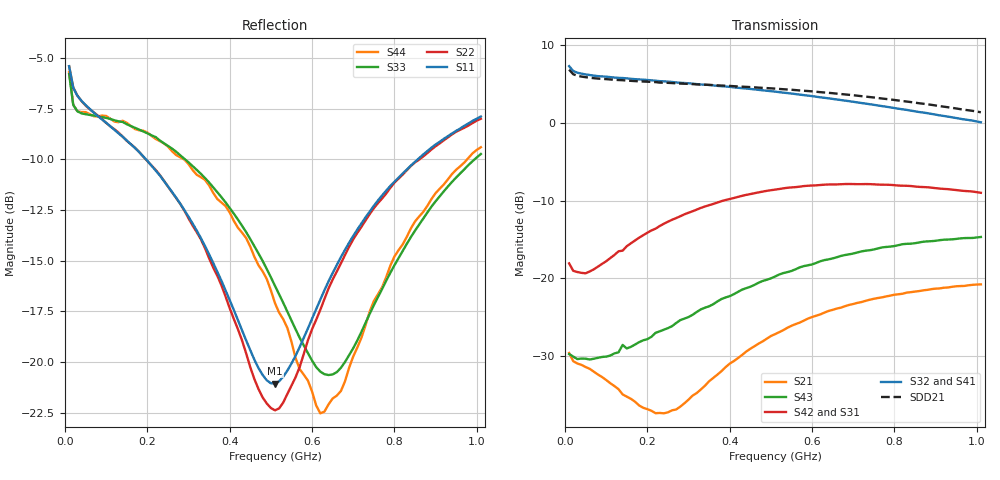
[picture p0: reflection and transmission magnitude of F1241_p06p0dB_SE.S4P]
! Integrated Device Technology
! Corporate Headquarters
! 6024 Silver Creek Valley Road
! San Jose, CA 95138  USA
! Phone:  1-408-284-8200
! Toll Free:  1-800-223-1366
! Webpage:  http://www.idt.com/
! Timing and RF Division
! 515 Groton Road, Suite 102
! Westford, MA 01886-6024
! Device:  F1241
! Description: Dual Intermediate Frequency Digital Variable Gain Amplifier
! Frequency:  10.0 -  500.00 MHz
! Package:  5x5 mm QFN Plastic Package: 32 pin
! Ports:  8 RF, 20 DC
!  Pin  1  = GA3  Pin 17  = RF OUT_B+
!  Pin  2  = GA4  Pin 18  = RF OUT_B-
!  Pin  3  = GA5  Pin 19  = STBY_B
!  Pin  4  = ISET_A  Pin 20  = Ground
!  Pin  5  = ISET_B  Pin 21  = Ground
!  Pin  6  = GB5  Pin 22  = STB_A
!  Pin  7  = GB4  Pin 23  = RF OUT_A-  = Port 4
!  Pin  8  = GB3  Pin 24  = RF OUT_A+  = Port 3
!  Pin  9  = GB2  Pin 25  = NO CONNECT
!  Pin 10  = GB1  Pin 26  = NO CONNECT
!  Pin 11  = RF IN_B+  Pin 27  = VCC
!  Pin 12  = RF IN_B-  Pin 28  = Ground
!  Pin 13  = Ground  Pin 29  = RF IN_A-  = Port 2
!  Pin 14  = VCC  Pin 30  = RF IN_A+  = Port 1
!  Pin 15  = NO CONNECT  Pin 31  = GA1
!  Pin 16  = NO CONNECT  Pin 32  = GA2
! State:  14
! Gain State:  6.0 dB
! Voltages:  Vcc = +5.00 Volts  Icc approximately 160.0 mA or 80 mA per channel.
! Data:  The device was measured on a custom evaluation board which has
!  individual transmission lines to the RF pins.  Data was collected
!  using a calibrated network analyzer.  The evaluation board was
!  de-embedded using a port reference technique.
!  The reference plane is the edge of the package pin.
!  Only Channel A was measured.
!  This data is in single-ended operation.  If your needs are balanced
!  or differential S-parameters then this file needs to be used a
!  linear simulator.
! Misc:  Lot Code  160028MY
!  Action Tracker AT004
! Date Measured:  2014-08-14
! Date:  2014-08-28  MJV
! Note:
!  Integrated Device Technology supplies this data as a sample of measured
!  data at the package pin for this product.  Your particular data for this
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# Hz S dB R 50
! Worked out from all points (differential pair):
!   101 points, 10 MHz to 1.01 GHz, reference 50 ohm
!   strongest paths, dB at 10 MHz, 260 MHz, 510 MHz, 760 MHz, 1.01 GHz:
!     S32: 7.3, 5.3, 4.0, 2.2, 0.1
!     S41: 7.3, 5.2, 4.0, 2.1, -0.1
!     S42: -18.1, -12.4, -8.6, -7.9, -9.0
!     S31: -18.0, -12.4, -8.6, -8.0, -9.1
!     S43: -29.7, -26.1, -19.8, -16.1, -14.7
!     S21: -29.6, -37.0, -27.2, -22.5, -20.8
!   taken as a pair (ports 2,1 in; 3,4 out), SDD21 dB: 6.9, 5.1, 4.4, 3.2, 1.4
!   lowest |S11| = -21.1 dB at 510 MHz (marker M1), VSWR 1.19, Z = 43.3 - j4.85 ohm
!   |S11| at or under -10 dB: 196.6 MHz to 856.8 MHz (660.2 MHz wide, 125 % of centre)
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1e7  -5.41 -20.5  -29.59 -23.2  -51.57 7.1  -17.51 14.6
     -29.59 -23.2  -5.41 -20.2  -17.53 14.3  -51.54 8.0
     -18.03 159.7  7.30 175.1  -5.78 -25.4  -29.86 -174.3
     7.33 175.2  -18.05 159.8  -29.71 -174.8  -5.70 -25.4
3e7  -6.86 -15.9  -30.96 -12.6  -49.25 40.8  -17.38 1.3
     -30.94 -12.5  -6.86 -15.6  -17.41 1.6  -49.42 40.7
     -19.16 145.1  6.47 171.7  -7.63 -12.7  -30.54 172.2
     6.50 171.6  -19.17 145.3  -30.37 172.2  -7.63 -12.3
1.1e8  -8.37 -24.7  -33.55 -12.5  -40.85 60.9  -17.75 -7.1
       -33.47 -13.2  -8.37 -23.3  -17.75 -7.3  -40.87 60.8
       -17.28 101.4  5.89 160.1  -8.01 -13.5  -29.99 156.6
       5.90 159.9  -17.37 102.0  -29.91 156.0  -8.00 -13.5
2.4e8  -11.06 -43.3  -36.92 27.4  -34.71 55.2  -17.84 -14.5
       -37.34 24.7  -11.05 -40.9  -17.79 -14.4  -34.68 54.1
       -12.88 63.5  5.35 141.8  -9.21 -26.4  -26.95 135.2
       5.33 141.2  -12.96 63.5  -26.59 134.4  -9.21 -25.0
5.1e8  -21.05 -141.2  -26.82 60.6  -29.17 32.8  -17.40 -33.1
       -27.16 62.9  -22.37 -140.1  -17.25 -32.8  -29.16 30.7
       -8.58 9.7  4.03 105.3  -16.24 -68.6  -20.14 97.6
       3.95 104.5  -8.57 8.7  -19.75 97.3  -17.09 -66.4
6.3e8  -16.46 157.8  -24.24 51.7  -27.79 23.1  -17.44 -42.9
       -24.39 55.1  -16.89 154.9  -17.21 -42.8  -27.77 20.0
       -7.99 -10.9  3.23 90.0  -20.59 -123.7  -18.15 81.4
       3.14 89.1  -7.94 -12.3  -17.64 80.1  -22.44 -129.2
1.01e9  -7.89 114.4  -20.91 24.3  -25.19 -8.3  -18.82 -72.6
        -20.76 26.1  -8.00 113.5  -18.31 -72.8  -25.26 -12.5
        -9.08 -61.5  0.08 47.8  -9.74 136.5  -15.08 34.9
        -0.09 47.1  -8.98 -64.5  -14.66 34.2  -9.40 132.1
